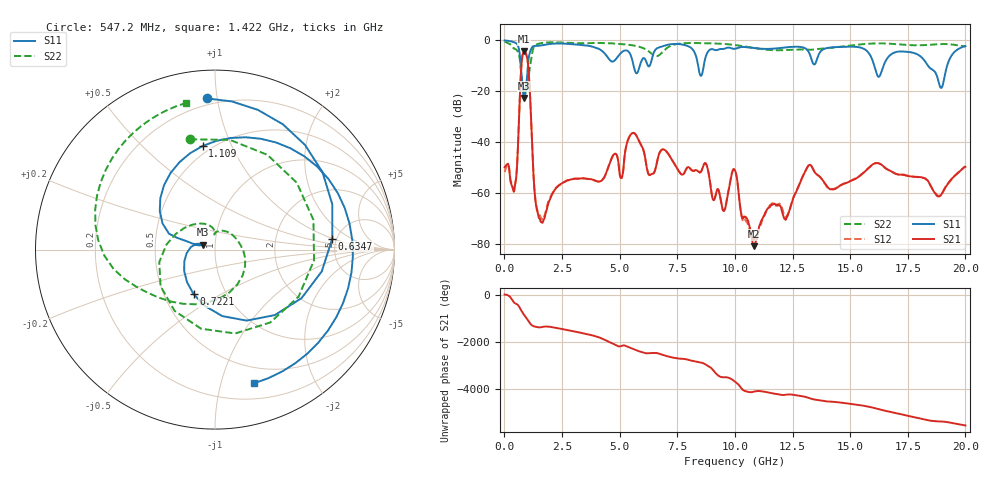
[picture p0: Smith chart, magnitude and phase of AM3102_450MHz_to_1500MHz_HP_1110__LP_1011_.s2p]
!Agilent Technologies,E8364B,MY43040894,A.07.50.67
!Agilent E8364B: A.07.50.67
!Date: Thursday, January 11, 2018 06:45:11
!Correction: S11(Full 2 Port(1,2))
!S21(Full 2 Port(1,2))
!S12(Full 2 Port(1,2))
!S22(Full 2 Port(1,2))
!S2P File: Measurements: S11, S21, S12, S22:
# Hz S  dB  R 50
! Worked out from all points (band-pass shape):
!   1601 points, 10 MHz to 20 GHz, reference 50 ohm
!   highest |S21| = -4.42 dB at 859.6 MHz (marker M1); lowest = -80.9 dB at 10.82 GHz (marker M2)
!   |S21| within 3 dB of the highest: 764.4 MHz to 996.5 MHz (232.1 MHz wide, 26.4 % of centre)
!   lowest |S11| = -22.7 dB at 859.6 MHz (marker M3), VSWR 1.16, Z = 43.6 + j2.47 ohm
!   |S11| at or under -10 dB: 710.4 MHz to 1.02 GHz (309.5 MHz wide, 35.8 % of centre); 16.05 GHz to 16.45 GHz (402.4 MHz wide, 2.48 % of centre); 18.38 GHz to 19.21 GHz (830.4 MHz wide, 4.42 % of centre)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
!   |S22| runs from -21.5 to -0.5 dB; largest |S21 - S12| = 0.00066
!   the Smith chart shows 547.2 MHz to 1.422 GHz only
!   S11 on the Smith chart (normalised r, x): 547.2 MHz: 0.16, +0.93; 634.7 MHz: 4.60, +0.99; 722.1 MHz: 0.70, -0.38; 1.109 GHz: 0.45, +0.78; 1.422 GHz: 0.34, -1.27
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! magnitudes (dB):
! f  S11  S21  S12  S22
! 10 MHz  -0.1  -49.9  -51.8  -0.5
! 397.3 MHz  -0.7  -59.4  -58.8  -3.1
! 547.2 MHz  -1.5  -49.8  -49.6  -4.0
! 634.7 MHz  -3.7  -30.5  -30.4  -5.9
! 722.1 MHz  -11.2  -12.1  -12.1  -12.6
! 859.6 MHz  -22.7  -4.4  -4.4  -21.3
! 1.109 GHz  -4.7  -20.8  -20.8  -10.5
! 1.422 GHz  -2.2  -67.1  -66.5  -1.6
! 3.346 GHz  -1.9  -54.3  -54.3  -1.2
! 5.082 GHz  -4.8  -54.1  -54.1  -1.5
! 5.57 GHz  -8.6  -36.4  -36.4  -2.0
! 6.294 GHz  -10.1  -53.0  -52.9  -4.6
! 6.682 GHz  -2.9  -45.5  -45.5  -6.1
! 8.731 GHz  -6.6  -48.4  -48.3  -1.2
! 9.518 GHz  -3.4  -67.1  -66.9  -1.5
! 10.01 GHz  -3.4  -51.1  -51.2  -1.9
! 10.82 GHz  -3.1  -80.9  -78.4  -3.0
! 13.34 GHz  -8.0  -49.7  -49.7  -3.7
! 14.22 GHz  -2.8  -58.6  -58.4  -2.9
! 16.68 GHz  -6.4  -51.0  -51.1  -1.3
! 18.95 GHz  -18.7  -60.7  -60.7  -1.5
! 20 GHz  -2.3  -49.7  -49.5  -2.5
